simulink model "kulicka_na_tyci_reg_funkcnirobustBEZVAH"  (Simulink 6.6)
settings: Solver=ode45  StartTime=0.0  StopTime=inf  FixedStep=0.01  RelTol=1e-3
undefined symbols (not defined in the file or in its folder): a, b, Humusoft, MF624, to, V
libraries: rtlib x4

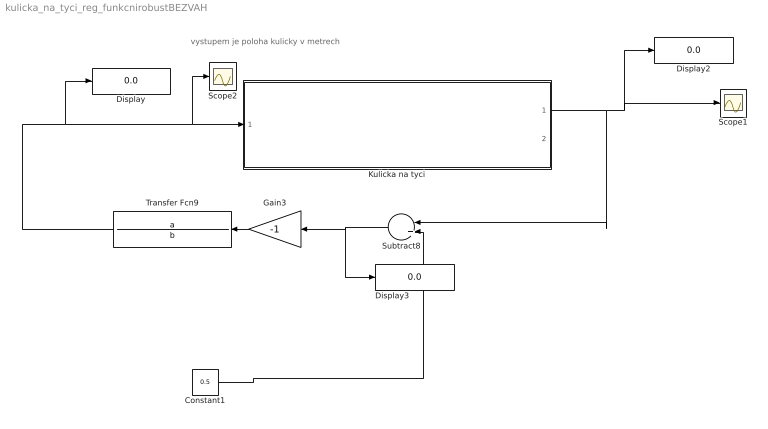
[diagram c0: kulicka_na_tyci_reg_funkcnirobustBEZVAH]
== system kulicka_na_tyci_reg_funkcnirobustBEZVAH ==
  note: vystupem je poloha kulicky v metrech
  Constant1 : Constant  Value=0.5
  Display : Display
  Display2 : Display
  Display3 : Display
  Gain3 : Gain  Orientation=left  Gain=-1
  Kulicka na tyci : Subsystem  TreatAsAtomicUnit=on  mask{Ts=0.02, IN_K=1, IN_R=2, OUT_S=1}
      mask prompts: Ts "Vzorkovaci perioda [s]"; IN_K "Cislo analog. vstupu - poloha kulicky"; IN_R "Cislo analog. vstupu - poloha ramane"; OUT_S "Cislo analog vystutpu - rizeni naklonu"
  Scope1 : Scope
  Scope2 : Scope
  Subtract8 : Sum  Orientation=left  Inputs=-+  OutScaling=2^-10
  Transfer Fcn9 : TransferFcn  Orientation=left  Numerator=a  Denominator=b
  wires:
  Kulicka na tyci/1(kulicka) -> Subtract8/1, Scope1/1, Display2/1
  Subtract8/1 -> Display3/1, Gain3/1
  Transfer Fcn9/1 -> Display/1, Kulicka na tyci/1(rameno), Scope2/1
  Constant1/1 -> Subtract8/2
  Gain3/1 -> Transfer Fcn9/1

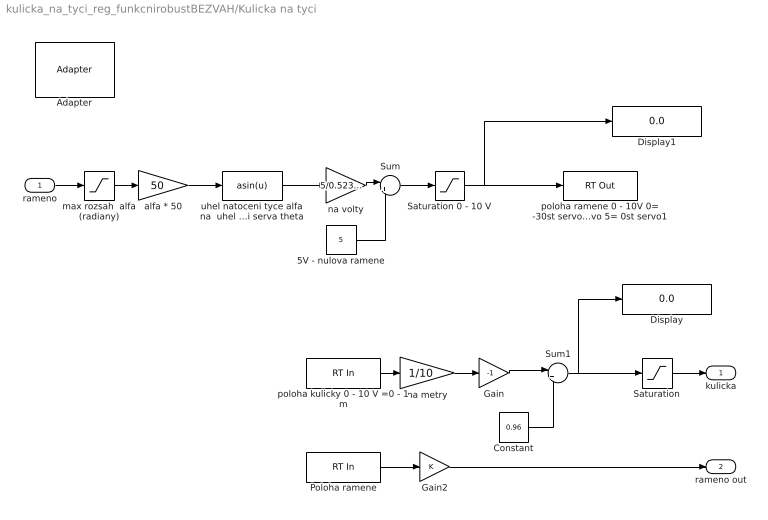
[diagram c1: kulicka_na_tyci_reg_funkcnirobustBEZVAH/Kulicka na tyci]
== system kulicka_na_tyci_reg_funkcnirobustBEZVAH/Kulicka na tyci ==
  rameno : Inport
  5V - nulova ramene : Constant  Value=5
  Adapter : rtlib/Adapter  SystemSampleTime=-1  DriverName=Humusoft/MF624  DriverAddress=4294967295  DriverOptions=0
  Constant : Constant  Value=0.96  SampleTime=-1
  Display : Display
  Display1 : Display
  Gain : Gain  Gain=-1
  Gain2 : Gain
  Poloha ramene : rtlib/RT In  SampleTime=Ts  Adapter=Adapter  IOClass=Analog Input  Channels=IN_R  SLDataType=double  MaxMissedTicks=100  ShowMissedTicks=off  YieldWhenWaiting=on  AIORange=-10 to 10 V  AIOUnits=Volts  DIOMode=Bit  CIReset=never  CIEdge=rising  CIGate=none  EIQuadrature=quadruple  EIIndexPulse=reset  EIFilterFrequency=Inf  OIOParameters=[]
  Saturation : Saturate  UpperLimit=0.95  LowerLimit=0
  Saturation 0 - 10 V : Saturate  UpperLimit=10  LowerLimit=0
  Sum : Sum  Inputs=|++
  Sum1 : Sum  Inputs=|++
  alfa * 50 : Gain  Gain=50
  max rozsah  alfa (radiany) : Saturate  UpperLimit=0.01  LowerLimit=-0.01
  na metry : Gain  Gain=1/10
  na volty : Gain  Gain=5/0.52359877559830
  poloha kulicky 0 - 10 V =0 - 1 m : rtlib/RT In  SampleTime=Ts  Adapter=Adapter  IOClass=Analog Input  Channels=IN_K  SLDataType=double  MaxMissedTicks=100  ShowMissedTicks=off  YieldWhenWaiting=on  AIORange=-10 to 10 V  AIOUnits=Volts  DIOMode=Bit  CIReset=never  CIEdge=rising  CIGate=none  EIQuadrature=quadruple  EIIndexPulse=reset  EIFilterFrequency=Inf  OIOParameters=[]
  poloha ramene 0 - 10V 0= -30st servo 10= +30st servo 5= 0st servo1 : rtlib/RT Out  SampleTime=Ts  Adapter=Adapter  IOClass=Analog Output  Channels=OUT_S  InitialValue=[0]  FinalValue=[0]  MaxMissedTicks=100  ShowMissedTicks=off  YieldWhenWaiting=on  AIORange=-10 to 10 V  AIOUnits=Volts  DIOMode=Bit  OIOParameters=[]
  uhel natoceni tyce alfa na  uhel natoceni serva theta : Fcn  Expr=asin(u)
  kulicka : Outport
  rameno out : Outport  Port=2
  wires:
  poloha kulicky 0 - 10 V =0 - 1 m/1 -> na metry/1
  rameno/1 -> max rozsah  alfa (radiany)/1
  Saturation 0 - 10 V/1 -> Display1/1, poloha ramene 0 - 10V 0= -30st servo 10= +30st servo 5= 0st servo1/1
  Poloha ramene/1 -> Gain2/1
  Gain2/1 -> rameno out/1
  uhel natoceni tyce alfa na  uhel natoceni serva theta/1 -> na volty/1
  alfa * 50/1 -> uhel natoceni tyce alfa na  uhel natoceni serva theta/1
  max rozsah  alfa (radiany)/1 -> alfa * 50/1
  na volty/1 -> Sum/1
  5V - nulova ramene/1 -> Sum/2
  Sum/1 -> Saturation 0 - 10 V/1
  na metry/1 -> Gain/1
  Saturation/1 -> kulicka/1
  Gain/1 -> Sum1/1
  Sum1/1 -> Saturation/1, Display/1
  Constant/1 -> Sum1/2
